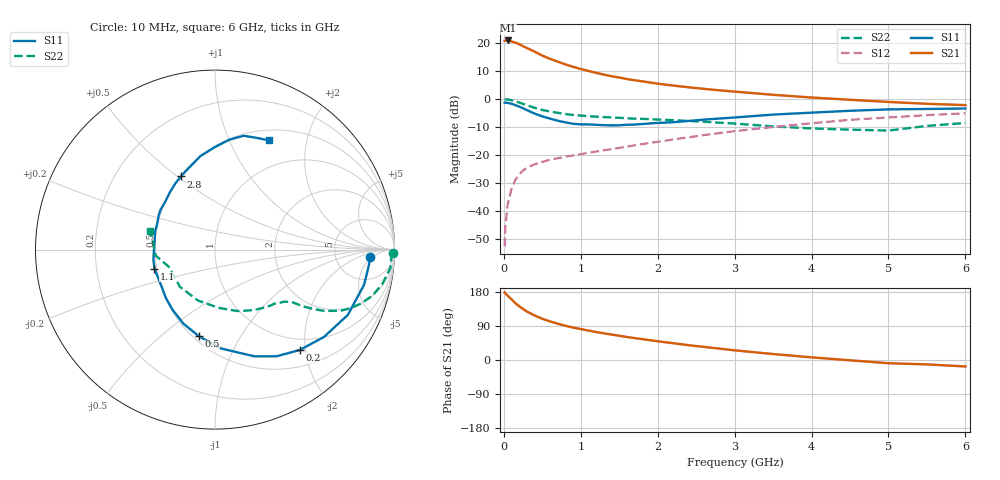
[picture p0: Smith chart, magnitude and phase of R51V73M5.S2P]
! SIEMENS Small Signal Semiconductors
! BFR183
! Si NPN RF Bipolar Junction Transistor in SOT23
! VCE = 1.75 V  IC = 3.5 mA
! Common Emitter S-Parameters:  May  1996
# GHz  S  MA  R  50
!  f  S11  S21  S12  S22
! GHz  MAG  ANG  MAG  ANG  MAG  ANG  MAG  ANG
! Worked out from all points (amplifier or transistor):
!   36 points, 10 MHz to 6 GHz, reference 50 ohm
!   highest |S21| = 20.9 dB at 50 MHz (marker M1)
!   |S21| within 3 dB of that: start of sweep to 323.8 MHz
!   unconditionally stable (mu >= 1): 1.174 GHz to 2.772 GHz
!   at 250 MHz: K = 0.33, MSG = 22.1 dB, |S12| = -25.4 dB
!   at 1.4 GHz: K = 1.07, MAG = 11.4 dB, |S12| = -17.8 dB
!   at 6 GHz: K = 0.90, MSG = 1.5 dB, |S12| = -5.1 dB
!   S11 on the Smith chart (normalised r, x): 10 MHz: 12, -4; 200 MHz: 0.79, -1.89; 500 MHz: 0.53, -0.68; 1.1 GHz: 0.49, -0.12; 2.8 GHz: 0.50, +0.52; 6 GHz: 0.63, +1.42
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0.01  0.8642 -2.7  10.89 178.3  0.0024 91.4  0.9921 -1.2
0.02  0.8623 -5.5  10.97 175.7  0.0053 87.2  0.9829 -2.3
0.05  0.8535 -13.3  11.03 169.6  0.0133 83.7  0.9824 -6.0
0.1  0.8246 -26.2  10.58 160.1  0.0252 76.9  0.9523 -11.5
0.15  0.7783 -38.7  10.12 149.8  0.0366 69.9  0.9132 -16.4
0.2  0.7321 -49.8  9.475 141.8  0.0455 65.1  0.8657 -20.4
0.25  0.6862 -60.0  8.721 134.5  0.0534 60.9  0.8193 -23.6
0.3  0.6335 -69.8  8.096 127.8  0.0598 58.1  0.7774 -26.0
0.4  0.5512 -86.7  6.968 117.5  0.0688 53.6  0.6982 -29.3
0.5  0.4908 -100.6  5.927 108.7  0.076 51.2  0.6381 -31.2
0.6  0.4483 -113.2  5.199 101.9  0.0831 49.8  0.6005 -32.3
0.7  0.4112 -124.8  4.63 95.8  0.0883 49.5  0.5684 -33.2
0.8  0.3843 -135.3  4.134 90.4  0.094 49.4  0.5417 -33.7
0.9  0.3627 -144.8  3.747 85.6  0.0991 50.2  0.5201 -34.3
1.1  0.3533 -162.6  3.161 77.7  0.1103 51.4  0.4947 -36.0
1.6  0.3486 163.7  2.268 60.7  0.1421 54.0  0.4541 -41.3
2.2  0.3863 135.4  1.736 44.3  0.1905 54.5  0.4202 -50.7
2.8  0.4495 115.0  1.429 30.1  0.247 51.6  0.3792 -63.9
3.5  0.5282 98.7  1.188 15.7  0.3173 45.0  0.3254 -86.3
4.5  0.6173 82.6  0.97 -0.8  0.4262 33.1  0.285 -133.3
5.5  0.6652 69.2  0.822 -11.6  0.5165 20.0  0.332 -174.3
6  0.6787 63.6  0.779 -17.1  0.5566 11.5  0.3748 163.8
